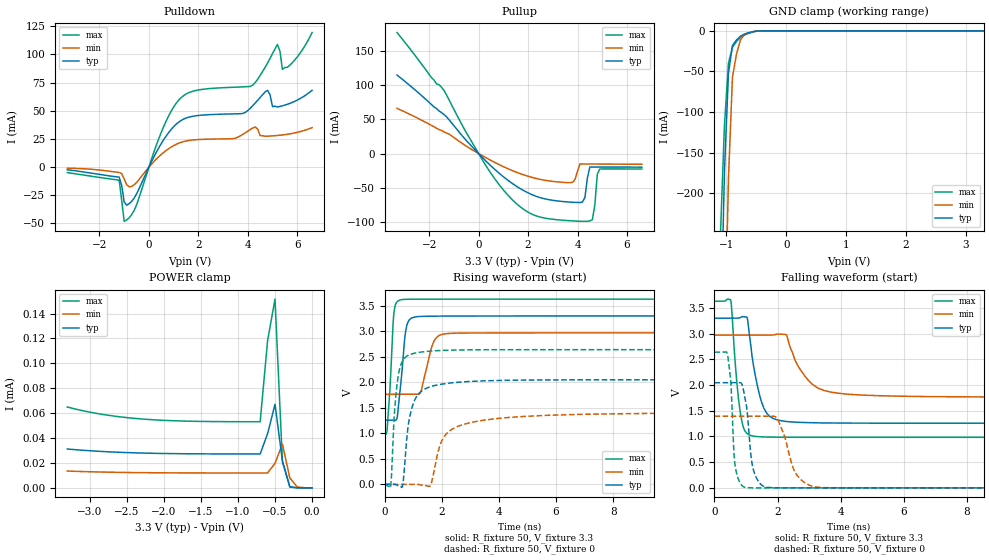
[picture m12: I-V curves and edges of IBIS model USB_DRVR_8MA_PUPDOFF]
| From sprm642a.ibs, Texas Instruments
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|   Model Cell USB_DRVR_8MA_PUPDOFF
|USB_DRVR_8MA_PUPDOFF
[Model]   USB_DRVR_8MA_PUPDOFF
Model_type   I/O
Polarity   Non-Inverting
Enable   Active-Low
Vinl =  0.8
Vinh =  2
Cref =  15.0000pF
Rref =  100.0000M
Vref =  0V
Vmeas =  1.65
C_comp   5.34973p   4.565931p   6.027791p
[Model Spec]
Vinl   0.8   0.8   0.8
Vinh   2   2   2
[Temperature Range]   25   155   -40
[Voltage Range]   3.3   2.97   3.63
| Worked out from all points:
|   slope of the pulldown table from 0 to 0.495 V, typ, clamps not added: 23.8 ohm
|   slope of the pullup table from 0 to 0.495 V, typ, clamps not added: 27.8 ohm
|   GND clamp passes 1 mA (typ) near -0.55 V on its own axis
|   rising waveform, R_fixture 50, V_fixture 3.3: 20-80 % time 202ps typ, 323ps min, 146ps max; typ from 1.26 V to 3.3 V
|   rising waveform, R_fixture 50, V_fixture 0: 20-80 % time 335ps typ, 753ps min, 202ps max; typ from 0 V to 2.04 V
|   falling waveform, R_fixture 50, V_fixture 3.3: 20-80 % time 369ps typ, 720ps min, 222ps max; typ from 3.3 V to 1.26 V
|   falling waveform, R_fixture 50, V_fixture 0: 20-80 % time 208ps typ, 431ps min, 126ps max; typ from 2.04 V to 0 V
| Nom Voltages:
|   BIASFET=3.3, VDD=1.2, VDDS=3.3, VSS=0
| Min Voltages:
|   BIASFET=2.97, VDD=1.08, VDDS=2.97, VSS=0
| Max Voltages:
|   BIASFET=3.63, VDD=1.32, VDDS=3.63, VSS=0
[POWER_clamp]
|   voltage   I(typ)   I(min)   I(max)
-3.3V     31.22uA    13.5uA     64.95uA
-2.8V     29.13uA    12.67uA    58.77uA
-2.3V     27.98uA    12.22uA    55.36uA
-1.7V     27.4uA     12.01uA    53.62uA
-700mV    27.24uA    11.95uA    53.12uA
-600mV    43.52uA    11.94uA    118.2uA
-500mV    67.21uA    19.79uA    151.6uA
-400mV    21.58uA    35.11uA    21.1uA
-300mV    927.4nA    7.959uA    611.4nA
-200mV    28.93nA    716.3nA    11.51nA
0V        696.9pA    39.48nA    568.3pA
[Pulldown]
|   voltage   I(typ)   I(min)   I(max)
-3.3V     -2.325mA   -885.1uA   -4.829mA
-1.2V     -8.9mA     -4.742mA   -11.78mA
-1V       -30.94mA   -10.56mA   -48.07mA
-900mV    -33.77mA   -15.53mA   -46.9mA
-500mV    -23.82mA   -13.61mA   -33.55mA
600mV     24.46mA    13.16mA    36.18mA
1.3V      41.39mA    22.04mA    61.62mA
4.2V      54.57mA    34.77mA    72.77mA
4.8V      68.22mA    27.49mA    92.41mA
5.2V      53.41mA    28.11mA    108.9mA
5.4V      54.46mA    28.58mA    86.79mA
6.6V      68.25mA    35.07mA    119.5mA
[Pullup]
|   voltage   I(typ)   I(min)   I(max)
-3.3V     114.4mA    65.88mA    176.4mA
-1.4V     56.91mA    31.53mA    92.06mA
700mV     -24.56mA   -13.78mA   -39.08mA
2V        -57.24mA   -33.05mA   -85.4mA
3.8V      -70.97mA   -41.82mA   -98.09mA
4.2V      -70.71mA   -15.14mA   -98.64mA
4.5V      -19.61mA   -15.2mA    -98.06mA
4.6V      -19.61mA   -15.22mA   -96.39mA
4.7V      -19.61mA   -15.23mA   -75.23mA
4.8V      -19.61mA   -15.26mA   -30.07mA
4.9V      -19.62mA   -15.28mA   -22.42mA
6.6V      -19.78mA   -15.6mA    -22.44mA
[GND_clamp]
|   voltage   I(typ)   I(min)   I(max)
-3.3V     -16.36A    -15.08A    -17.18A
-1.1V     -382.1mA   -717.8mA   -250.1mA
-1.033V   -173.3mA   -402.2mA   -116.4mA
-966.7mV  -52.02mA   -182.1mA   -39.81mA
-900mV    -18.21mA   -57.43mA   -20.34mA
-833.3mV  -11.36mA   -28.88mA   -13.17mA
-766.7mV  -6.618mA   -11.27mA   -8.134mA
-700mV    -3.983mA   -4.59mA    -5.247mA
-500mV    -328.3uA   -481.4uA   -374.5uA
-366.7mV  -15.94uA   -50.74uA   -14.83uA
3.3V      696.9pA    15.85uA    426.1pA
[Ramp]
| variable   typ   min   max
dV/dt_f  1.2435216/0.37043762n 0.73534822/0.72019621n  1.6127085/0.22297403n
dV/dt_r  1.2644443/0.33444283n 0.86590685/0.74181111n  1.6251292/0.20296461n
R_load = 50
[Rising Waveform]
R_fixture = 50
V_fixture = 3.3
V_fixture_min = 2.97
V_fixture_max = 3.63
|   time   V(typ)   V(min)   V(max)
0s        1.258V     1.765V     982.5mV
85.2ps    1.258V     1.765V     1.096V
315.7ps   1.257V     1.765V     3.333V
437.8ps   1.319V     1.765V     3.583V
542.5ps   1.871V     1.765V     3.615V
758.1ps   3.083V     1.765V     3.627V
1.108ns   3.285V     1.763V     3.629V
1.723ns   3.297V     2.804V     3.629V
2.171ns   3.298V     2.954V     3.63V
20.04ns   3.3V       2.97V      3.63V
[Rising Waveform]
R_fixture = 50
V_fixture = 0
V_fixture_min = 0
V_fixture_max = 0
|   time   V(typ)   V(min)   V(max)
0s        0V         0V         0V
207.3ps   0V         0V         -33.86mV
380.1ps   -2.907mV   0V         1.694V
612.5ps   -47.07mV   0V         2.41V
825.9ps   1.176V     0V         2.53V
1.059ns   1.664V     0V         2.573V
1.594ns   1.913V     -24.86mV   2.612V
2.235ns   1.983V     1.033V     2.629V
3.521ns   2.029V     1.262V     2.638V
20.01ns   2.045V     1.397V     2.639V
[Falling Waveform]
R_fixture = 50
V_fixture = 3.3
V_fixture_min = 2.97
V_fixture_max = 3.63
|   time   V(typ)   V(min)   V(max)
0s        3.3V       2.97V      3.63V
514.8ps   3.3V       2.97V      3.65V
832.2ps   3.317V     2.97V      1.409V
1.039ns   3.301V     2.97V      1.055V
1.229ns   2.405V     2.97V      1.007V
1.652ns   1.454V     2.97V      988.1mV
2.329ns   1.288V     2.889V     983.7mV
3.102ns   1.266V     2.015V     982.8mV
4.108ns   1.26V      1.828V     982.7mV
20.04ns   1.258V     1.765V     982.8mV
[Falling Waveform]
R_fixture = 50
V_fixture = 0
V_fixture_min = 0
V_fixture_max = 0
|   time   V(typ)   V(min)   V(max)
0s        2.045V     1.393V     2.639V
415.4ps   2.045V     1.393V     2.583V
520.2ps   2.045V     1.393V     2.031V
650.1ps   2.045V     1.393V     457.4mV
953.8ps   1.791V     1.393V     11.73mV
1.226ns   369mV      1.393V     0V
1.663ns   10.2mV     1.394V     0V
2.643ns   0V         225.6mV    0V
3.336ns   0V         7.273mV    0V
20.01ns   0V         0V         0V
